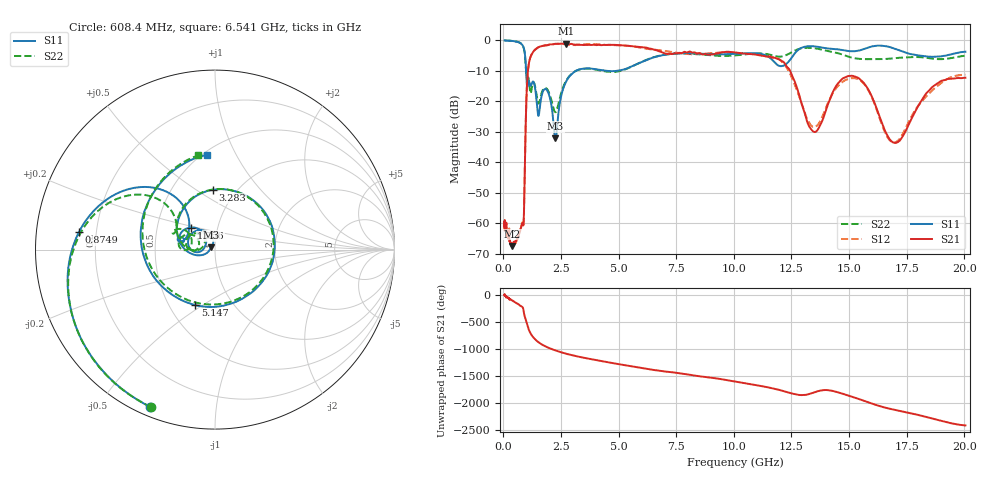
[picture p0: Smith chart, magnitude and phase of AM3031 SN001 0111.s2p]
# Hz S DB R 50
!freq MagS11 AngS11 MagS21 AngS21 MagS12 AngS12 MagS22 AngS22
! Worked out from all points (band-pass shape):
!   1601 points, 50 MHz to 20.05 GHz, reference 50 ohm
!   highest |S21| = -1.05 dB at 2.702 GHz (marker M1); lowest = -67.5 dB at 385.2 MHz (marker M2)
!   |S21| within 3 dB of the highest: 1.264 GHz to 6.924 GHz (5.659 GHz wide, 138 % of centre); 9.395 GHz to 10.17 GHz (778 MHz wide, 7.95 % of centre)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
!   lowest |S11| = -32.2 dB at 2.257 GHz (marker M3), VSWR 1.05, Z = 47.9 + j1.19 ohm
!   |S11| at or under -10 dB: 982.1 MHz to 3.135 GHz (2.153 GHz wide, 105 % of centre); 4.503 GHz to 4.895 GHz (392.7 MHz wide, 8.36 % of centre)
!   |S22| runs from -23.6 to 0.0 dB; largest |S21 - S12| = 0.067
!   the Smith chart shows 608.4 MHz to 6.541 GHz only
!   S11 on the Smith chart (normalised r, x): 608.4 MHz: 0.04, -0.67; 874.9 MHz: 0.13, +0.06; 1.356 GHz: 0.75, +0.19; 3.283 GHz: 0.78, +0.59; 5.147 GHz: 0.67, -0.47; 6.541 GHz: 0.53, +0.77
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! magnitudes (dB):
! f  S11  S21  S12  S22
! 50 MHz  0.0  -59.6  -62.5  0.0
! 135.9 MHz  -0.1  -62.9  -62.6  0.0
! 369.6 MHz  -0.2  -67.1  -67.4  -0.2
! 385.2 MHz  -0.2  -67.5  -67.1  -0.2
! 608.4 MHz  -0.5  -65.2  -65.0  -0.5
! 874.9 MHz  -2.3  -59.8  -59.7  -2.4
! 1.005 GHz  -13.4  -17.3  -17.2  -12.0
! 1.356 GHz  -14.9  -3.1  -3.2  -14.5
! 1.518 GHz  -24.7  -2.2  -2.2  -20.7
! 1.929 GHz  -16.9  -1.5  -1.5  -16.4
! 2.257 GHz  -32.2  -1.1  -1.2  -23.6
! 2.702 GHz  -13.8  -1.1  -1.3  -13.5
! 2.722 GHz  -13.5  -1.1  -1.3  -13.2
! 3.283 GHz  -9.5  -1.4  -1.4  -9.6
! 5.147 GHz  -9.7  -1.6  -1.6  -9.9
! 6.541 GHz  -5.5  -3.0  -3.0  -5.5
! 7.402 GHz  -4.3  -4.3  -4.0  -4.3
! 11.87 GHz  -7.9  -6.0  -5.9  -5.3
! 13.48 GHz  -1.9  -30.0  -28.4  -2.5
! 15.2 GHz  -3.6  -11.7  -12.4  -5.8
! 16.94 GHz  -2.6  -33.6  -33.6  -5.8
! 20.05 GHz  -3.7  -12.2  -11.2  -5.0
